FUNCTION "ALARM_MAN" : VOID
TITLE =EXCHANGE DATA         LINE <-> PRESS          MANAGEMENT
AUTHOR : DM
VERSION : 0.1

BEGIN
NETWORK
TITLE =SIGNAL TO PRESS
//STEP POSITION OK              E21.2 INGRESSO GESTITO DALL'ABB (NON DALLA FM354)
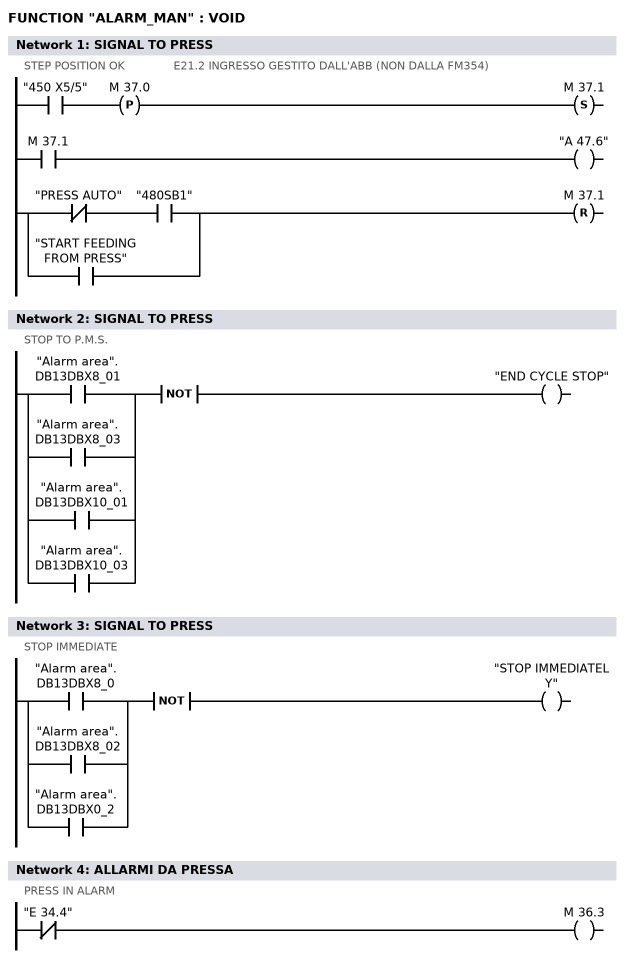
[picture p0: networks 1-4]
      U     "450 X5/5";
      FP    M     37.0;
      S     M     37.1;

      U     M     37.1;
      =     "A      47.6";

      UN    "PRESS AUTO";
      U     "480SB1";
      O     "START FEEDING FROM PRESS";
      R     M     37.1;
NETWORK
TITLE =SIGNAL TO PRESS
//STOP TO P.M.S.
      O     "Alarm area".DB13DBX8_01;
      O     "Alarm area".DB13DBX8_03;
      O     "Alarm area".DB13DBX10_01;
      O     "Alarm area".DB13DBX10_03;
      NOT   ;
      =     "END CYCLE STOP";
NETWORK
TITLE =SIGNAL TO PRESS
//STOP IMMEDIATE
      O     "Alarm area".DB13DBX8_0;
      O     "Alarm area".DB13DBX8_02;
      O     "Alarm area".DB13DBX0_2;
      NOT   ;
      =     "STOP IMMEDIATELY";
NETWORK
TITLE =ALLARMI DA PRESSA
//PRESS IN ALARM
      UN    "E      34.4";
      =     M     36.3;

END_FUNCTION

